FUNCTION_BLOCK FB_LN_IED_LD1_LEDGGIO6 EXTENDS FB_AcsiCommonLogicalNodeClass
VAR_INPUT
	NamPlt: FB_DO_IED_LD1_LEDGGIO6_NamPlt := (sClass:='LPL', bLinkResult:=THIS^.AddDataToContainer(ipData:=NamPlt));
	Beh: FB_DO_IED_LD1_LEDGGIO6_Beh := (sClass:='ENS', bLinkResult:=THIS^.AddDataToContainer(ipData:=Beh));
	Health: FB_DO_IED_LD1_LEDGGIO6_Health := (sClass:='ENS', bLinkResult:=THIS^.AddDataToContainer(ipData:=Health));
	Mod_: FB_DO_IED_LD1_LEDGGIO6_Mod := (sObjectName:='Mod', sClass:='ENC', bLinkResult:=THIS^.AddDataToContainer(ipData:=Mod_));
	SPCSO1: FB_DO_IED_LD1_LEDGGIO6_SPCSO1 := (sClass:='SPC', bLinkResult:=THIS^.AddDataToContainer(ipData:=SPCSO1));
END_VAR
VAR
END_VAR

END_FUNCTION_BLOCK
